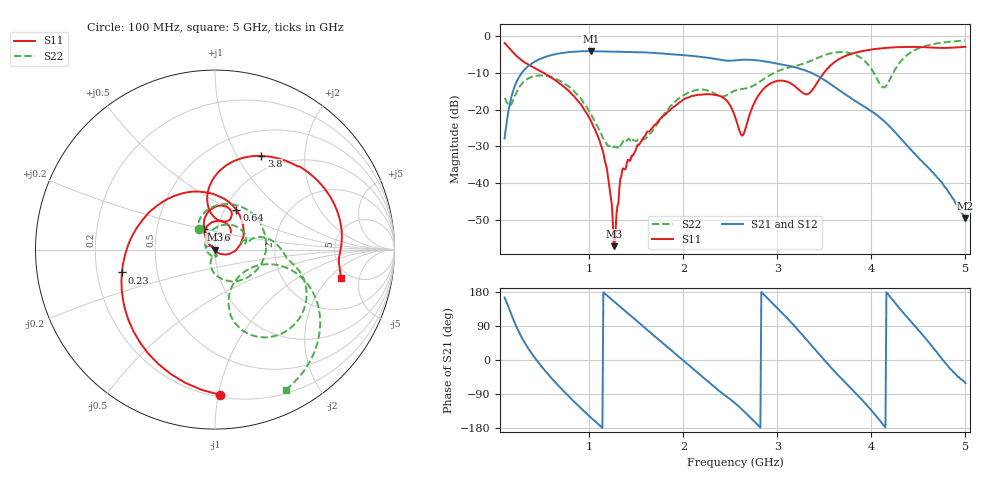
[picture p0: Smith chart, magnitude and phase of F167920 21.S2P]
!  2-Port S-parameters saved by WinCal
! VAR MeasName=S-Parameters (CALIBRATED_DATA) read from VNA (N5242A)
! VAR MeasDate=2016-11-22 9:56:13
! VAR NAME=F167920 21
! VAR FILENAME=F167920 21.S2P
! VAR DATE=2016-11-22 9:56:13
! VAR PHYS_PORTS=1,2
# Hz S DB R 50
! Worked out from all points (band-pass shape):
!   491 points, 100 MHz to 5 GHz, reference 50 ohm
!   highest |S21| = -4.07 dB at 1.02 GHz (marker M1); lowest = -49.6 dB at 5 GHz (marker M2)
!   |S21| within 3 dB of the highest: 410.8 MHz to 2.918 GHz (2.507 GHz wide, 151 % of centre)
!   lowest |S11| = -57.2 dB at 1.26 GHz (marker M3), VSWR 1.00, Z = 49.9 - j0.105 ohm
!   |S11| at or under -10 dB: 514.5 MHz to 3.495 GHz (2.98 GHz wide, 149 % of centre)
!   |S22| runs from -30.7 to -1.2 dB; largest |S21 - S12| = 0.0012
!   S11 on the Smith chart (normalised r, x): 100 MHz: 0.22, -1.01; 230 MHz: 0.31, -0.11; 640 MHz: 1.14, +0.54; 2.76 GHz: 0.87, +0.20; 3.8 GHz: 0.80, +1.27; 5 GHz: 4.24, -2.75
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1e8  -1.83 -87.9  -27.89 164.8  -27.89 164.8  -16.81 128.4
2.3e8  -5.45 -166.2  -12.26 85.4  -12.26 85.5  -15.10 121.5
4.4e8  -8.95 117.2  -6.64 -0.3  -6.64 -0.4  -10.75 40.4
6.4e8  -12.01 61.6  -4.89 -59.2  -4.89 -59.2  -11.58 -22.1
9.2e8  -18.78 -3.1  -4.08 -129.1  -4.09 -129.1  -17.29 -91.3
1.02e9  -23.16 -23.3  -4.07 -152.5  -4.08 -152.5  -21.37 -107.0
1.17e9  -34.37 -51.0  -4.16 174.3  -4.16 174.3  -28.84 -102.8
1.26e9  -57.24 -130.3  -4.23 155.1  -4.23 155.1  -30.09 -83.4
1.35e9  -36.59 143.2  -4.23 135.9  -4.23 135.9  -29.15 -71.5
1.74e9  -22.93 132.3  -4.65 53.4  -4.65 53.4  -23.37 140.5
2.07e9  -16.55 99.5  -5.32 -15.9  -5.32 -15.9  -15.16 48.4
2.4e9  -16.41 57.6  -6.46 -85.2  -6.46 -85.2  -16.37 11.5
2.55e9  -21.88 40.2  -6.58 -113.8  -6.58 -113.8  -14.82 16.0
2.63e9  -27.09 82.1  -6.41 -131.7  -6.41 -131.7  -14.38 13.6
2.76e9  -17.92 118.0  -6.51 -163.3  -6.51 -163.4  -13.29 16.2
3.09e9  -12.28 71.5  -7.90 114.3  -7.91 114.3  -8.75 1.1
3.37e9  -14.72 92.2  -10.06 36.4  -10.07 36.4  -6.57 -12.8
3.8e9  -4.70 63.7  -17.16 -78.8  -17.20 -78.8  -4.79 -57.7
4.02e9  -3.55 43.0  -20.76 -138.2  -20.80 -138.0  -9.74 -76.3
4.19e9  -3.12 29.4  -24.47 169.5  -24.50 169.7  -12.09 -21.5
4.5e9  -2.94 8.2  -33.12 78.9  -33.10 79.0  -3.33 -31.3
5e9  -2.88 -12.7  -49.61 -61.2  -49.94 -59.3  -1.15 -63.3
